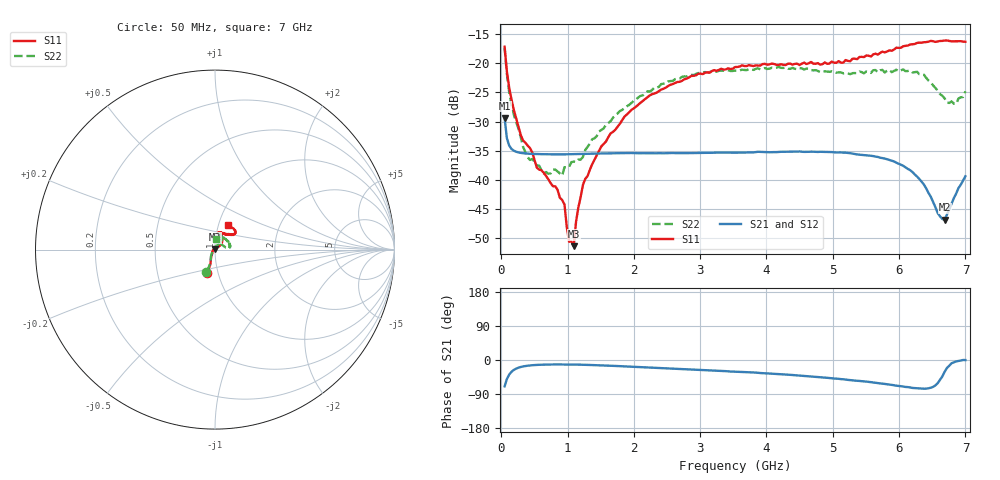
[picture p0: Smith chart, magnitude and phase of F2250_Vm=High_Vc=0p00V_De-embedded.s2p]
! Integrated Device Technology
! Corporate Headquarters
! 6024 Silver Creek Valley Road
! San Jose, CA 95138  USA
! Phone:  1-408-284-8200
! Toll Free:  1-800-223-1366
! Webpage:  http://www.idt.com/
! Timing and RF Division
! 515 Groton Road, Suite 102
! Westford, MA 01886-6024
! Device:  F2250
! Description: Voltage Variable RF Attenuator
! Frequency:  50.0 -  6000.00 MHz
! Package:  3x3 mm Thin QFN Plastic Package: 16 pin
! Ports:  2 RF, 3 DC
!  Pin  1  = GND
!  Pin  2  = NC
!  Pin  3  = RF1  = Port 1
!  Pin  4  = NC
!  Pin  5  = GND
!  Pin  6  = GND
!  Pin  7  = GND
!  Pin  8  = GND
!  Pin  9  = NC
!  Pin 10  = RF2  = Port 2
!  Pin 11  = NC
!  Pin 12  = GND
!  Pin 13  = GND
!  Pin 14  = VCNTRL
!  Pin 15  = VDD
!  Pin 16  = VMODE
! Vcntrl:  0.000 Volts
! Vmode:  +3.300 Volts
! Vdd:  +3.30  Volts
! Current:  1.244 mA
! Data:  The device was measured on a the F2250 evaluation board which has
!  individual transmission lines to the RF pins.  Data was collected
!  using a calibrated network analyzer.  The evaluation board was
!  de-embedded using a TRL calibration technique.
!  The reference plane is the edge of the package pin.
! Misc:  SN 10
!  Action Tracker AT0258
! Date Measured:  2014-11-26
! Date:  2015-10-15  MJV
! Note:
!  Integrated Device Technology supplies this data as a sample of measured
!  data at the package pin for this product.  Your particular data for this
!  product may vary.
!  Data was taken at 25 degrees C.
!  Integrated Device Technology reserves the right to change this data at anytime.
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# GHz S dB R 50
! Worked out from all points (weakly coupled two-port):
!   201 points, 50 MHz to 7 GHz, reference 50 ohm
!   highest |S21| = -29.38 dB at 50 MHz (marker M1); lowest = -46.8 dB at 6.687 GHz (marker M2)
!   lowest |S11| = -51.3 dB at 1.093 GHz (marker M3), VSWR 1.01, Z = 50 + j0.271 ohm
!   |S11| at or under -10 dB: start of sweep to end of sweep
!   |S22| runs from -39.2 to -17.4 dB; largest |S21 - S12| = 6e-05
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0.05  -17.18 -108.5  -29.38 -69.5  -29.38 -69.5  -17.37 -110.5
0.08475  -21.47 -107.4  -32.86 -50.1  -32.86 -50.1  -21.87 -109.0
0.15425  -26.22 -116.6  -34.68 -31.0  -34.68 -31.0  -27.10 -120.7
0.29325  -32.27 -127.4  -35.35 -18.5  -35.35 -18.4  -32.66 -133.6
0.3975  -34.10 -142.3  -35.48 -15.0  -35.48 -15.0  -36.08 -158.3
0.5365  -37.90 -154.6  -35.55 -13.0  -35.55 -12.9  -37.51 179.9
0.64075  -38.77 -162.7  -35.58 -12.2  -35.58 -12.2  -38.88 160.4
0.91875  -43.42 156.2  -35.60 -11.8  -35.60 -11.8  -39.23 127.9
0.9535  -44.20 170.9  -35.60 -11.8  -35.60 -11.8  -37.79 124.1
1.023  -50.58 139.9  -35.59 -11.9  -35.59 -11.9  -37.73 108.1
1.0925  -51.33 89.5  -35.57 -12.0  -35.57 -12.0  -36.84 98.7
1.12725  -47.16 61.6  -35.56 -12.1  -35.56 -12.1  -36.92 91.7
1.2315  -40.84 40.9  -35.52 -12.4  -35.52 -12.5  -36.05 77.2
1.6485  -32.02 41.2  -35.44 -15.2  -35.44 -15.2  -29.92 59.9
2.37825  -24.76 46.7  -35.40 -21.0  -35.40 -21.0  -24.03 53.9
3.525  -20.65 71.7  -35.32 -30.6  -35.32 -30.6  -21.26 73.0
4.7065  -20.06 72.0  -35.15 -43.9  -35.15 -43.9  -21.21 70.4
5.85325  -17.79 40.5  -36.58 -64.8  -36.58 -64.9  -21.13 23.4
6.305  -16.47 40.4  -39.82 -75.3  -39.83 -75.4  -21.87 8.5
6.68725  -16.11 47.9  -46.81 -31.0  -46.80 -30.7  -26.02 28.5
6.861  -16.22 54.5  -42.31 -3.7  -42.27 -3.8  -26.95 57.4
7  -16.32 62.4  -39.36 -0.1  -39.33 -0.2  -24.81 83.6
